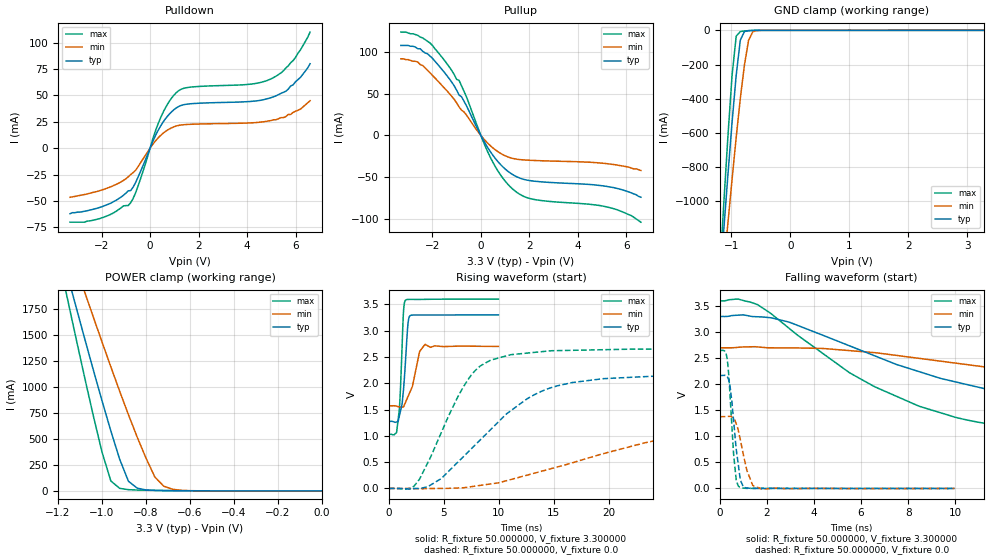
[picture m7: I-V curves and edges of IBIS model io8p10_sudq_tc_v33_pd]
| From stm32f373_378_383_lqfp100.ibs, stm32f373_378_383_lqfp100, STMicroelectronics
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|   Model io8p10_sudq_tc_v33_pd
[Model]  io8p10_sudq_tc_v33_pd
Model_type I/O
Polarity   Non-Inverting
Enable   Active-Low
Vinl =   0.990000V
Vinh =   2.310000V
Vmeas =  1.650000V
Cref =   50.000000pF
Rref =   100.000000M
Vref =   0.0V
C_comp   1.325200pF   1.251200pF   1.426700pF
[Temperature Range]   25.000000   0.125000k   -40.000000
[Pullup Reference]   3.300000V   2.700000V   3.600000V
[Pulldown Reference]   0.0V   0.0V   0.0V
[POWER Clamp Reference]   3.300000V   2.700000V   3.600000V
[GND Clamp Reference]   0.0V   0.0V   0.0V
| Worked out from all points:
|   slope of the pulldown table from 0 to 0.495 V, typ, clamps not added: 21.3 ohm
|   slope of the pullup table from 0 to 0.495 V, typ, clamps not added: 20.9 ohm
|   GND clamp passes 1 mA (typ) near -0.66 V on its own axis
|   POWER clamp passes 1 mA (typ) near -0.60 V on its own axis
|   rising waveform, R_fixture 50.000000, V_fixture 3.300000: 20-80 % time 415ps typ, 825ps min, 303ps max; typ from 1.27 V to 3.3 V
|   rising waveform, R_fixture 50.000000, V_fixture 0.0: 20-80 % time 6.86ns typ, 16.4ns min, 3.73ns max; typ from 0 V to 2.17 V
|   falling waveform, R_fixture 50.000000, V_fixture 3.300000: 20-80 % time 9.32ns typ, 15.5ns min, 5.81ns max; typ from 3.3 V to 1.27 V
|   falling waveform, R_fixture 50.000000, V_fixture 0.0: 20-80 % time 298ps typ, 421ps min, 225ps max; typ from 2.17 V to 0 V
[Pulldown]
|Voltage   I(typ)   I(min)   I(max)
-3.3V     -62mA      -46.4mA    -70mA
-2.1V     -56.2mA    -40.3mA    -66.8mA
-800mV    -40.04mA   -24.9mA    -51.58mA
-500mV    -27.57mA   -17.6mA    -36.07mA
400mV     19.71mA    11.36mA    27.01mA
700mV     29.83mA    16.93mA    40.97mA
1.1V      38.46mA    21.2mA     53.02mA
1.6V      41.98mA    22.62mA    57.7mA
4.1V      44.26mA    24mA       60.59mA
5V        48mA       26.3mA     65.8mA
5.9V      60mA       34mA       83mA
6.6V      80mA       45mA       110mA
[Pullup]
|Voltage   I(typ)   I(min)   I(max)
-3.3V     108mA      92mA       124mA
-2.6V     104mA      88mA       120mA
-2.2V     98mA       78.2mA     113mA
-1.4V     71.8mA     53.6mA     86.1mA
-900mV    48.51mA    34.23mA    66.14mA
-700mV    41.33mA    28.36mA    53.31mA
400mV     -19.77mA   -12.52mA   -26.8mA
900mV     -37.48mA   -22.89mA   -50.99mA
1.4V      -48.39mA   -28.06mA   -66.43mA
2.2V      -54.79mA   -29.98mA   -76.75mA
5.3V      -61.7mA    -34.2mA    -86.4mA
6.6V      -74mA      -42mA      -104mA
[GND_clamp]
|Voltage   I(typ)   I(min)   I(max)
-3.3V     -9.739A    -9.975A    -9.587A
-1.2V     -1.489A    -1.65A     -1.416A
-1.13V    -1.162A    -1.385A    -1.009A
-1.06V    -842.3mA   -1.125A    -616.9mA
-990mV    -537.1mA   -870.2mA   -263mA
-920mV    -262.5mA   -625.3mA   -33.98mA
-850mV    -56.96mA   -397.5mA   -7.097mA
-780mV    -7.026mA   -202.3mA   -3.727mA
-710mV    -1.792mA   -58.24mA   -1.753mA
-640mV    -564.1uA   -8.795mA   -558.4uA
-570mV    -123.3uA   -1.303mA   -102.2uA
3.28V     84.11uA    64.12uA    93.81uA
[POWER_clamp]
|Voltage   I(typ)   I(min)   I(max)
-3.28V    9.897A     9.838A     9.594A
-1.16V    2.103A     2.419A     1.88A
-1.12V    1.788A     2.17A      1.488A
-1.08V    1.476A     1.923A     1.102A
-1V       868.1mA    1.435A     373.1mA
-960mV    578.2mA    1.196A     96.06mA
-880mV    93.24mA    734.1mA    12.01mA
-840mV    26.3mA     517.4mA    8.56mA
-760mV    5.106mA    134mA      5.119mA
-720mV    3.355mA    46.34mA    3.808mA
-600mV    1.005mA    2.564mA    1.072mA
0V        0A         0A         0A
[Ramp]
| variable   typ   min   max
dV/dt_r  1.29948/6.85503n   0.81090/16.47332n   1.58814/3.72436n
dV/dt_f  1.21488/9.31457n   0.67002/15.56164n   1.54218/5.80049n
R_load = 50.000000
[Rising Waveform]
R_fixture= 50.000000
V_fixture= 3.300000
V_fixture_min= 2.700000
V_fixture_max= 3.600000
|time   V(typ)   V(min)   V(max)
0s        1.274V     1.569V     1.029V
720.7ps   1.264V     1.562V     1.093V
961ps     1.382V     1.55V      1.515V
1.201ns   1.602V     1.547V     2.683V
1.341ns   1.9V       1.553V     3.391V
1.502ns   2.38V      1.63V      3.574V
1.842ns   3.256V     1.794V     3.592V
2.803ns   3.296V     2.603V     3.592V
3.283ns   3.295V     2.737V     3.593V
9.97ns    3.299V     2.699V     3.599V
[Rising Waveform]
R_fixture= 50.000000
V_fixture= 0.0
V_fixture_min= 0.0
V_fixture_max= 0.0
|time   V(typ)   V(min)   V(max)
0s        1.008nV    9.499nV    1.541nV
2.302ns   -1.482mV   -3.505mV   46.05mV
4.705ns   179.7mV    24.27uV    1.03V
7.407ns   734mV      31.18mV    2.129V
9.209ns   1.108V     83.83mV    2.433V
11.01ns   1.465V     164.5mV    2.537V
14.61ns   1.905V     367.5mV    2.614V
19.52ns   2.086V     662mV      2.636V
31.53ns   2.157V     1.171V     2.647V
49.85ns   2.166V     1.377V     2.647V
[Falling Waveform]
R_fixture= 50.000000
V_fixture= 3.300000
V_fixture_min= 2.700000
V_fixture_max= 3.600000
|time   V(typ)   V(min)   V(max)
0s        3.299V     2.699V     3.599V
1.602ns   3.294V     2.715V     3.527V
2.903ns   3.196V     2.696V     3.088V
5.506ns   2.737V     2.644V     2.222V
8.408ns   2.249V     2.499V     1.589V
12.21ns   1.812V     2.283V     1.188V
15.82ns   1.554V     2.099V     1.086V
20.62ns   1.385V     1.911V     1.048V
35.24ns   1.279V     1.623V     1.03V
49.85ns   1.274V     1.569V     1.029V
[Falling Waveform]
R_fixture= 50.000000
V_fixture= 0.0
V_fixture_min= 0.0
V_fixture_max= 0.0
|time   V(typ)   V(min)   V(max)
0s        2.166V     1.377V     2.647V
320.3ps   2.143V     1.381V     2.467V
440.4ps   1.954V     1.383V     1.777V
600.6ps   1.254V     1.341V     610.4mV
700.7ps   756.9mV    1.24V      166.3mV
840.8ps   284.1mV    1.008V     27.15mV
1.001ns   30.44mV    655.9mV    6.788mV
1.401ns   1.976mV    60.12mV    956.2uV
1.802ns   447.6uV    -12.32mV   1.032mV
9.97ns    1.008nV    9.499nV    1.541nV
